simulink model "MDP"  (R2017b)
settings: Solver=FixedStepDiscrete  StartTime=0.0  StopTime=10.0  FixedStep=0.01  RelTol=1e-3  EnableMultiTasking=on
undefined symbols (not defined in the file): ASWTYPE_FALSE, ASWTYPE_TRUE
libraries: AIWAYS_Powertrain_BMS_lib x7

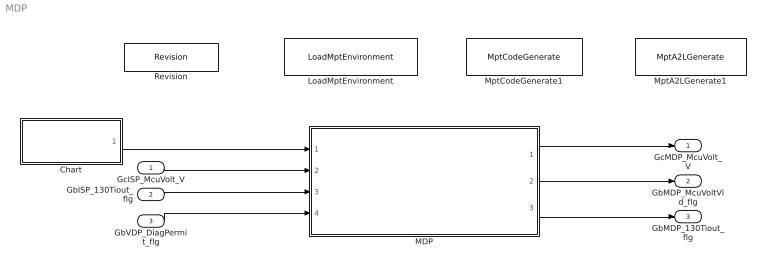
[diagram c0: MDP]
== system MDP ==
  GcISP_McuVolt_V : Inport
  GbISP_130Tiout_flg : Inport  Port=2
  GbVDP_DiagPermit_flg : Inport  Port=3
  Chart : Stateflow chart  TreatAsAtomicUnit=on
  LoadMptEnvironment : AIWAYS_Powertrain_BMS_lib/Config/LoadMptEnvironment  ProjectName=Comm  SuppierID=NewPlatformUAES
  MDP : Subsystem
  MptA2LGenerate1 : AIWAYS_Powertrain_BMS_lib/Config/MptA2LGenerate  SystemSampleTime=-1
  MptCodeGenerate1 : AIWAYS_Powertrain_BMS_lib/Config/MptCodeGenerate  SystemSampleTime=-1
  Revision : AIWAYS_Powertrain_BMS_lib/Config/Revision  curVersion='M100C100'  newVersion='M100C100'
  GcMDP_McuVolt_V : Outport
  GbMDP_McuVoltVld_flg : Outport  Port=2
  GbMDP_130Tiout_flg : Outport  Port=3
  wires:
  Chart/1(MDP_McuDataPrc_10ms()) -> MDP/1(MDP_McuDataPrc_10ms)
  GcISP_McuVolt_V/1 -> MDP/2(GcISP_McuVolt_V)
  GbISP_130Tiout_flg/1 -> MDP/3(GbISP_130Tiout_flg)
  MDP/1(GcMDP_McuVolt_V) -> GcMDP_McuVolt_V/1
  MDP/2(GbMDP_McuVoltVld_flg) -> GbMDP_McuVoltVld_flg/1
  GbVDP_DiagPermit_flg/1 -> MDP/4(GbVDP_DiagPermit_flg)
  MDP/3(GbMDP_130Tiout_flg) -> GbMDP_130Tiout_flg/1

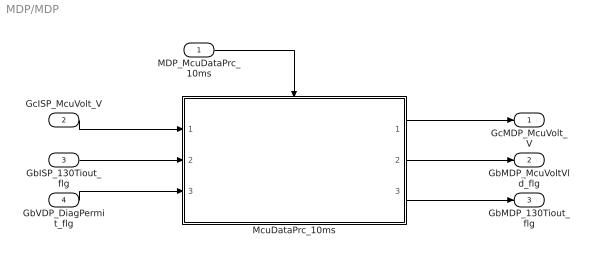
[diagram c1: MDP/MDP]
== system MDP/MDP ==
  MDP_McuDataPrc_10ms : Inport
  GcISP_McuVolt_V : Inport  Port=2
  GbISP_130Tiout_flg : Inport  Port=3
  GbVDP_DiagPermit_flg : Inport  Port=4
  McuDataPrc_10ms : Subsystem
  GcMDP_McuVolt_V : Outport
  GbMDP_McuVoltVld_flg : Outport  Port=2
  GbMDP_130Tiout_flg : Outport  Port=3
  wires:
  MDP_McuDataPrc_10ms/1 -> McuDataPrc_10ms/Trigger
  GcISP_McuVolt_V/1 -> McuDataPrc_10ms/1(GcISP_McuVolt_V)
  GbISP_130Tiout_flg/1 -> McuDataPrc_10ms/2(GbISP_130Tiout_flg)
  McuDataPrc_10ms/1(GcMDP_McuVolt_V) -> GcMDP_McuVolt_V/1
  McuDataPrc_10ms/2(GbMDP_McuVoltVld_flg) -> GbMDP_McuVoltVld_flg/1
  GbVDP_DiagPermit_flg/1 -> McuDataPrc_10ms/3(GbVDP_DiagPermit_flg)
  McuDataPrc_10ms/3(GbMDP_130Tiout_flg) -> GbMDP_130Tiout_flg/1

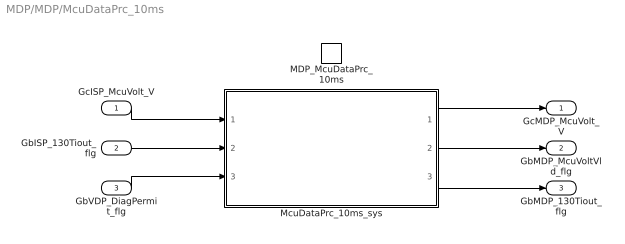
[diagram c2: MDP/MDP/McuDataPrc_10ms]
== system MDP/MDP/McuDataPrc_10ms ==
  GcISP_McuVolt_V : Inport
  GbISP_130Tiout_flg : Inport  Port=2
  GbVDP_DiagPermit_flg : Inport  Port=3
  MDP_McuDataPrc_10ms : TriggerPort  TriggerType=function-call  VariantControl=(inherit)
  McuDataPrc_10ms_sys : Subsystem
  GcMDP_McuVolt_V : Outport
  GbMDP_McuVoltVld_flg : Outport  Port=2
  GbMDP_130Tiout_flg : Outport  Port=3
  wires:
  GcISP_McuVolt_V/1 -> McuDataPrc_10ms_sys/1(GcISP_McuVolt_V)
  GbISP_130Tiout_flg/1 -> McuDataPrc_10ms_sys/2(GbISP_130Tiout_flg)
  McuDataPrc_10ms_sys/1(GcMDP_McuVolt_V) -> GcMDP_McuVolt_V/1
  McuDataPrc_10ms_sys/2(GbMDP_McuVoltVld_flg) -> GbMDP_McuVoltVld_flg/1
  GbVDP_DiagPermit_flg/1 -> McuDataPrc_10ms_sys/3(GbVDP_DiagPermit_flg)
  McuDataPrc_10ms_sys/3(GbMDP_130Tiout_flg) -> GbMDP_130Tiout_flg/1

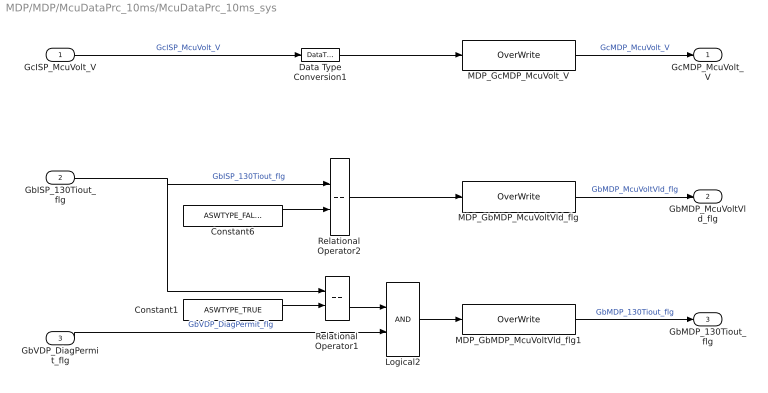
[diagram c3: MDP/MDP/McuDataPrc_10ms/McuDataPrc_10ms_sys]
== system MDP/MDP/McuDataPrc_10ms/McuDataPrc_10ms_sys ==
  GcISP_McuVolt_V : Inport
  GbISP_130Tiout_flg : Inport  Port=2
  GbVDP_DiagPermit_flg : Inport  Port=3
  Constant1 : Constant  Value=ASWTYPE_TRUE
  Constant6 : Constant  Value=ASWTYPE_FALSE
  Data Type Conversion1 : DataTypeConversion
  Logical2 : Logic  OutDataTypeStr=boolean
  MDP_GbMDP_McuVoltVld_flg : AIWAYS_Powertrain_BMS_lib/Signals/OverWrite  OverWrite_Value=CbMDP_McuVoltVldOvr_flg  OverWrite_flag=CbMDP_McuVoltVldOvrSwt_flg
  MDP_GbMDP_McuVoltVld_flg1 : AIWAYS_Powertrain_BMS_lib/Signals/OverWrite  OverWrite_Value=CbMDP_130TioutOvr_flg  OverWrite_flag=CbMDP_130TioutOvrSwt_flg
  MDP_GcMDP_McuVolt_V : AIWAYS_Powertrain_BMS_lib/Signals/OverWrite  OverWrite_Value=CcMDP_McuVoltOvr_V  OverWrite_flag=CbMDP_McuVoltOvrSwt_flg
  Relational Operator1 : RelationalOperator  Operator===  OutDataTypeStr=boolean
  Relational Operator2 : RelationalOperator  Operator===  OutDataTypeStr=boolean
  GcMDP_McuVolt_V : Outport
  GbMDP_McuVoltVld_flg : Outport  Port=2
  GbMDP_130Tiout_flg : Outport  Port=3
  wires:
  Constant6/1 -> Relational Operator2/2
  GbISP_130Tiout_flg/1 -> Relational Operator1/1, Relational Operator2/1  "GbISP_130Tiout_flg"
  Relational Operator2/1 -> MDP_GbMDP_McuVoltVld_flg/1
  GcISP_McuVolt_V/1 -> Data Type Conversion1/1  "GcISP_McuVolt_V"
  MDP_GbMDP_McuVoltVld_flg/1 -> GbMDP_McuVoltVld_flg/1  "GbMDP_McuVoltVld_flg"
  Data Type Conversion1/1 -> MDP_GcMDP_McuVolt_V/1
  MDP_GcMDP_McuVolt_V/1 -> GcMDP_McuVolt_V/1  "GcMDP_McuVolt_V"
  Constant1/1 -> Relational Operator1/2
  GbVDP_DiagPermit_flg/1 -> Logical2/2  "GbVDP_DiagPermit_flg"
  Relational Operator1/1 -> Logical2/1
  Logical2/1 -> MDP_GbMDP_McuVoltVld_flg1/1
  MDP_GbMDP_McuVoltVld_flg1/1 -> GbMDP_130Tiout_flg/1  "GbMDP_130Tiout_flg"

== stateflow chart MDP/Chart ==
  (default) -> (junction 1)
  (junction 1) -> (junction 3) : {MDP_McuDataPrc_10ms;}
  events: output FUNCTION_CALL_EVENT
